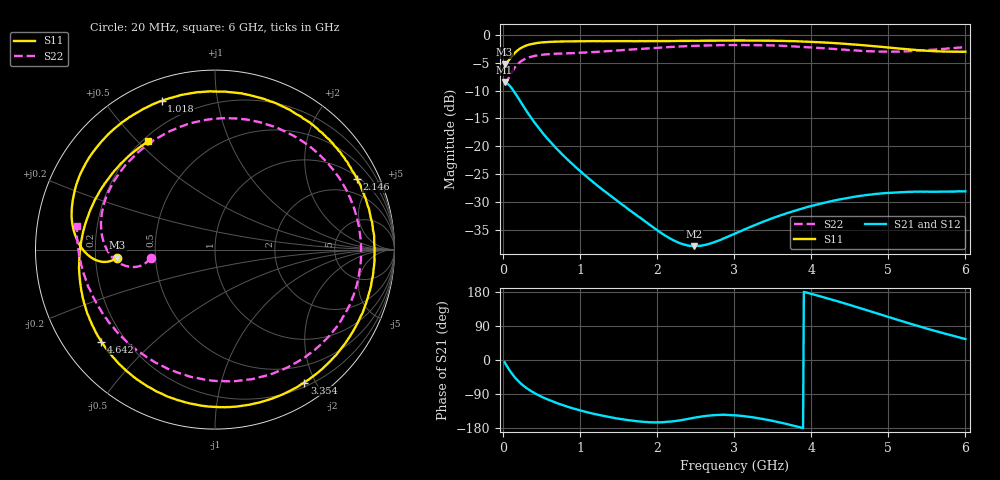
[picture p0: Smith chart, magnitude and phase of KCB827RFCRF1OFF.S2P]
!Agilent Technologies,E5071B,JP1KK00126,A.08.11
!Date: Tue May 06 07:38:01 2014
!Data & Calibration Information:
!Freq	S11:SOLT2(ON)	S21:SOLT2(ON)	S12:SOLT2(ON)	S22:SOLT2(ON)
# Hz S dB R 50
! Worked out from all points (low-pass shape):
!   600 points, 20 MHz to 6 GHz, reference 50 ohm
!   highest |S21| = -8.43 dB at 20 MHz (marker M1); lowest = -38.0 dB at 2.476 GHz (marker M2)
!   |S21| within 3 dB of the highest: start of sweep to 201.9 MHz
!   lowest |S11| = -5.2 dB at 20 MHz (marker M3), VSWR 3.41, Z = 14.7 - j1.85 ohm
!   |S11| at or under -10 dB: nowhere
!   |S22| runs from -8.9 to -1.8 dB; largest |S21 - S12| = 0.00071
!   S11 on the Smith chart (normalised r, x): 20 MHz: 0.29, -0.04; 1.018 GHz: 0.10, +0.70; 2.146 GHz: 1.10, +3.96; 3.354 GHz: 0.25, -1.85; 4.642 GHz: 0.11, -0.35; 6 GHz: 0.22, +0.54
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2e7  -5.24 -175.4  -8.43 -5.9  -8.43 -5.9  -8.89 -172.8
1.597663e8  -3.10 -176.9  -10.51 -47.4  -10.50 -47.3  -5.71 -170.5
2.795659e8  -1.99 172.1  -13.14 -70.3  -13.13 -70.3  -4.33 179.1
4.093489e8  -1.50 159.8  -15.76 -87.6  -15.74 -87.5  -3.74 167.6
7.088481e8  -1.17 134.1  -20.64 -114.4  -20.63 -114.4  -3.34 145.0
1.018331e9  -1.11 109.8  -24.69 -133.9  -24.69 -134.0  -3.18 123.3
1.247947e9  -1.09 92.3  -27.35 -145.0  -27.35 -145.0  -3.00 107.7
1.497529e9  -1.09 73.7  -30.01 -154.9  -29.99 -154.7  -2.76 90.7
1.777062e9  -1.07 53.2  -32.84 -162.4  -32.85 -162.2  -2.48 71.5
2.016661e9  -1.08 35.9  -35.28 -164.4  -35.26 -164.5  -2.27 55.4
2.146444e9  -1.07 26.5  -36.44 -163.1  -36.46 -162.9  -2.15 47.2
2.475893e9  -1.03 3.3  -38.00 -152.6  -38.00 -152.5  -1.93 27.5
2.735459e9  -0.99 -14.7  -37.30 -145.5  -37.30 -145.6  -1.83 12.8
3.014992e9  -0.98 -33.7  -35.69 -146.2  -35.69 -146.1  -1.78 -2.2
3.354424e9  -0.99 -56.1  -33.70 -155.0  -33.73 -155.0  -1.81 -19.4
3.693856e9  -1.07 -78.2  -32.01 -169.6  -32.02 -169.7  -1.96 -37.2
4.013322e9  -1.22 -98.8  -30.71 173.8  -30.70 173.9  -2.23 -55.6
4.322805e9  -1.46 -119.3  -29.71 156.0  -29.71 156.1  -2.53 -75.5
4.64227e9  -1.78 -141.0  -28.93 136.4  -28.94 136.4  -2.82 -98.5
5.011653e9  -2.25 -167.1  -28.40 112.9  -28.38 113.0  -2.98 -126.7
5.440935e9  -2.76 161.6  -28.19 86.3  -28.18 86.5  -2.78 -157.7
6e9  -2.99 121.6  -28.13 55.1  -28.14 55.4  -2.15 170.5
